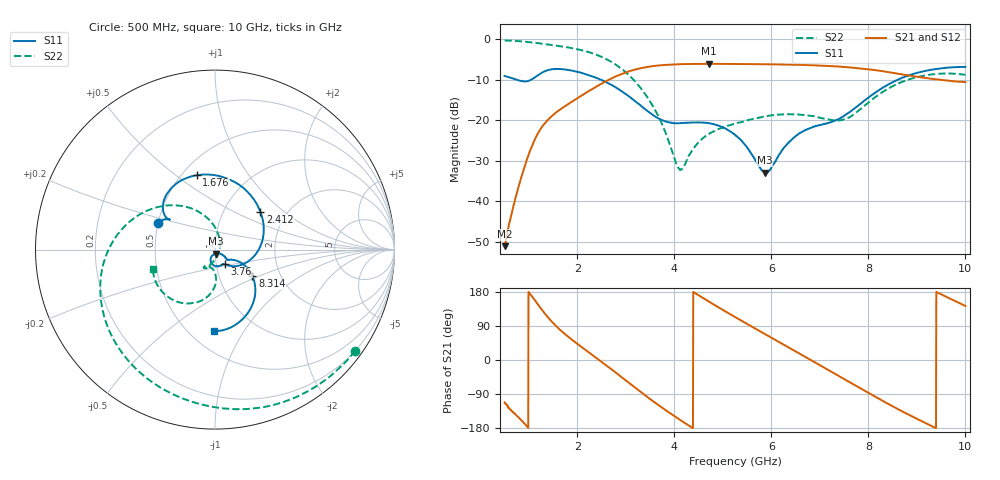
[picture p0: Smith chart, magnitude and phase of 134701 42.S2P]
!  2-Port S-parameters saved by WinCal
! VAR MeasName=S-Parameters (CALIBRATED_DATA) read from VNA (N5242A)
! VAR MeasDate=2013-7-3 16:37:54
! VAR NAME=134701 42
! VAR FILENAME=134701 42.S2P
! VAR DATE=2013-7-3 16:37:54
! VAR PHYS_PORTS=1,2
# Hz S MA R 50
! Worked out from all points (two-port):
!   1601 points, 500 MHz to 10 GHz, reference 50 ohm
!   highest |S21| = -6.08 dB at 4.716 GHz (marker M1); lowest = -51.0 dB at 500 MHz (marker M2)
!   |S21| within 3 dB of the highest: 2.811 GHz to 8.902 GHz (6.091 GHz wide, 104 % of centre)
!   lowest |S11| = -32.9 dB at 5.867 GHz (marker M3), VSWR 1.05, Z = 50.3 - j2.24 ohm
!   |S11| at or under -10 dB: 747.4 MHz to 1.048 GHz (301 MHz wide, 33.5 % of centre); 2.484 GHz to 8.606 GHz (6.121 GHz wide, 110 % of centre)
!   |S22| runs from -32.2 to -0.3 dB; largest |S21 - S12| = 0.0022
!   S11 on the Smith chart (normalised r, x): 500 MHz: 0.50, +0.17; 1.676 GHz: 0.59, +0.60; 2.412 GHz: 1.48, +0.70; 3.76 GHz: 1.10, -0.18; 8.314 GHz: 1.44, -0.46; 10 GHz: 0.65, -0.75
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5e8  0.352 155.3  0.002814 -111.8  0.00289 -113.2  0.963 -35.9
7.909375e8  0.3105 146.6  0.01547 -151.9  0.01539 -152.4  0.9439 -56.5
1.07e9  0.3217 147.0  0.04916 166.8  0.0491 166.6  0.9112 -76.3
1.343125e9  0.4054 132.7  0.09426 120.2  0.09407 120.1  0.8659 -94.9
1.675625e9  0.4267 103.9  0.1397 75.8  0.1394 75.7  0.813 -117.2
2.085312e9  0.3843 68.9  0.2016 34.5  0.2011 34.5  0.7312 -146.0
2.411875e9  0.3292 39.9  0.2648 3.8  0.2642 3.9  0.6362 -170.6
2.987812e9  0.2125 -13.0  0.387 -52.8  0.3871 -52.6  0.3955 143.0
3.338125e9  0.1462 -39.4  0.4426 -87.5  0.4428 -87.4  0.2358 114.5
3.670625e9  0.106 -53.3  0.4737 -118.9  0.4736 -118.9  0.112 86.5
3.759688e9  0.09993 -55.4  0.4786 -127.0  0.4789 -127.0  0.08592 77.4
4.121875e9  0.09202 -62.8  0.4906 -158.4  0.4906 -158.4  0.0245 -13.1
4.715625e9  0.09192 -88.1  0.4965 153.9  0.4959 153.9  0.06815 -98.5
5.25e9  0.06633 -112.0  0.4944 113.5  0.4945 113.5  0.09118 -108.4
5.8675e9  0.02258 -80.0  0.49 68.5  0.4903 68.5  0.1117 -114.4
6.401875e9  0.05645 -35.0  0.4855 29.8  0.4853 29.8  0.1186 -120.5
6.835312e9  0.08151 -39.1  0.4773 -1.8  0.4776 -1.7  0.113 -122.4
7.524062e9  0.1162 -29.5  0.4531 -52.0  0.4533 -52.0  0.1036 -101.6
8.31375e9  0.2555 -35.4  0.4011 -109.2  0.4017 -109.2  0.2272 -93.0
8.420625e9  0.2778 -38.5  0.3919 -116.7  0.3919 -116.7  0.2481 -96.2
9.133125e9  0.4014 -63.7  0.3351 -163.7  0.3357 -163.6  0.3541 -123.9
1e10  0.4548 -90.6  0.2956 142.5  0.2965 142.7  0.363 -162.6
